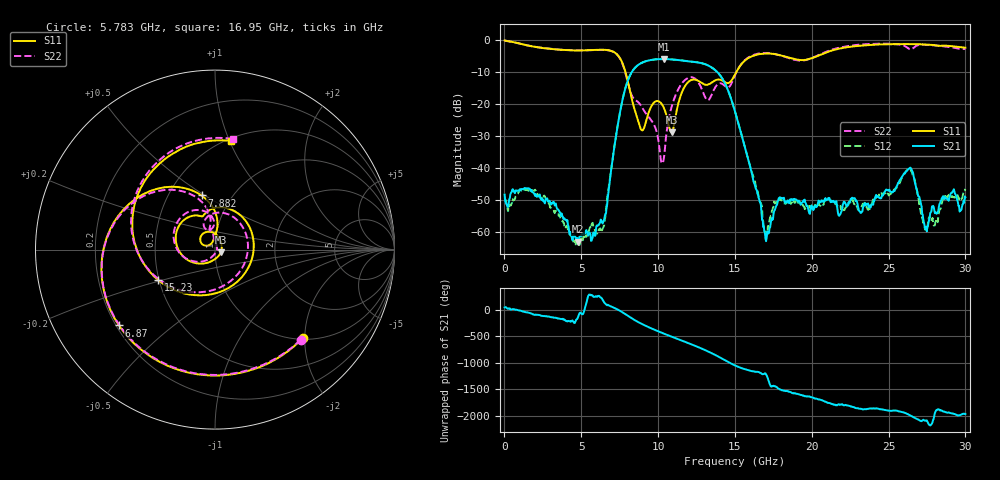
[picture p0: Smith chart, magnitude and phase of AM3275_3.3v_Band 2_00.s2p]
!Keysight Technologies,N5245B,MY58422270,A.16.20.02
!Date: Thursday, March 27, 2025 01:50:44
!Correction: S11(C  2-Port  )
!S21(C  2-Port  )
!S12(C  2-Port  )
!S22(C  2-Port  )
!S2P File: Measurements: S11, S21, S12, S22:
# Hz S  dB  R 50
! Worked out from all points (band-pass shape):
!   801 points, 10 MHz to 30 GHz, reference 50 ohm
!   highest |S21| = -5.98 dB at 10.36 GHz (marker M1); lowest = -63.0 dB at 4.808 GHz (marker M2)
!   |S21| within 3 dB of the highest: 8.446 GHz to 13.59 GHz (5.146 GHz wide, 46.7 % of centre)
!   lowest |S11| = -28.9 dB at 10.88 GHz (marker M3), VSWR 1.07, Z = 53.4 - j1.58 ohm
!   |S11| at or under -10 dB: 7.873 GHz to 15.09 GHz (7.221 GHz wide, 62.9 % of centre)
!   |S22| runs from -38.5 to -0.2 dB; largest |S21 - S12| = 0.0038
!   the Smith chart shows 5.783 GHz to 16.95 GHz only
!   S11 on the Smith chart (normalised r, x): 5.783 GHz: 1.03, -1.96; 6.87 GHz: 0.21, -0.33; 7.882 GHz: 0.73, +0.48; 15.23 GHz: 0.49, -0.19; 16.95 GHz: 0.52, +1.01
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1e7  -0.18 -5.9  -48.29 41.9  -49.21 6.8  -0.21 -6.5
8.34725e8  -0.97 -85.4  -47.08 -3.4  -48.14 -9.8  -0.99 -85.3
1.95935e9  -2.14 -171.3  -48.31 -96.5  -47.09 -91.2  -2.16 -171.4
4.8084e9  -3.33 23.2  -62.99 -124.6  -63.58 -82.2  -3.26 22.1
5.033325e9  -3.31 8.6  -60.71 -83.3  -61.95 -111.4  -3.27 7.4
5.783075e9  -3.17 -45.1  -60.08 -115.6  -58.30 -106.9  -3.19 -46.5
6.870212e9  -3.33 -141.7  -43.58 70.0  -43.05 74.3  -3.37 -142.1
7.882375e9  -10.16 103.9  -14.84 -86.4  -14.84 -86.5  -10.52 108.2
9.007e9  -28.15 134.8  -7.00 82.3  -6.99 82.2  -21.43 96.9
1.001916e10  -19.12 119.6  -6.02 -48.1  -6.02 -48.2  -31.31 70.4
1.035655e10  -21.05 90.1  -5.98 -87.9  -5.98 -87.9  -37.51 -50.1
1.088138e10  -28.89 -24.3  -6.09 -147.8  -6.08 -147.9  -20.85 -134.7
1.193102e10  -13.29 172.5  -6.66 95.2  -6.65 95.2  -11.92 152.5
1.331806e10  -13.81 107.6  -8.13 -74.9  -8.12 -75.0  -18.58 110.7
1.5005e10  -10.78 -120.2  -22.33 30.8  -22.31 30.7  -11.06 -123.2
1.522992e10  -8.89 -151.8  -26.10 2.9  -26.14 2.8  -8.87 -154.3
1.695435e10  -4.26 81.8  -60.35 -116.2  -59.68 -91.0  -4.08 80.8
1.841636e10  -5.40 -5.7  -50.11 -92.1  -50.43 -89.2  -5.53 -9.3
2.002832e10  -5.67 -135.6  -52.24 149.6  -51.96 144.7  -5.61 -139.9
2.246501e10  -2.20 104.8  -50.74 -11.3  -50.52 -28.5  -1.85 104.8
2.501416e10  -1.35 38.4  -47.04 -99.9  -48.58 -99.2  -1.20 35.9
3e10  -2.43 -109.8  -49.07 -162.1  -46.49 -151.5  -2.83 -108.7
